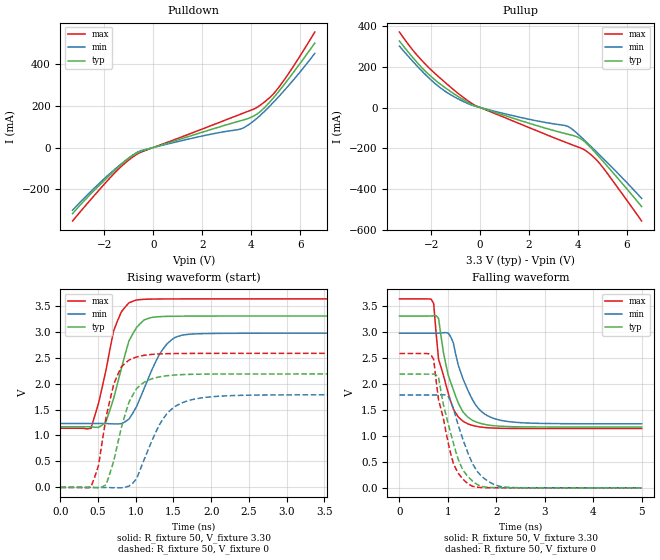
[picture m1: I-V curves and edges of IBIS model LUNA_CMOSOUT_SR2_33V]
[IBIS Ver]   3.2
[Comment Char]   |_char
[File name]   sg8201cja_33v_c.ibs
[File Rev]   1.1
[Date]   2021/10/19 9:35:58
[Source]
[Notes]
[Disclaimer]
This information is for modeling purposes only, and is not guaranteed.
Property of SEIKO EPSON Corp.,
unauthorized reproduction and/or distribution is strictly prohibited.
[Copyright]
Copyright 2021, SEIKO EPSON Corp.
[Component]   2G005_2016
Si_location Pin
Timing_location Pin
[Manufacturer]   SEIKO EPSON Corp.
| 2016 PKG
[Package]
R_pkg   25m   NA   NA
L_pkg   0.25n   NA   NA
C_pkg   0.183p   NA   NA
[Pin] signal_name   model_name
1   OE   NC
2   GND   GND
3   OUT   LUNA_CMOSOUT_SR2_33V
4   VCC   POWER
| Models and submodels in the file (1): LUNA_CMOSOUT_SR2_33V (Output)
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[Model]   LUNA_CMOSOUT_SR2_33V
Model_type Output
Polarity Non-Inverting
Vmeas=1.65
C_comp   2.5p   2.0p   3.0p
[Temperature Range] 25   140   -40
[Voltage Range]   3.30   2.97   3.63
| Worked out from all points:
|   slope of the pulldown table from 0 to 0.495 V, typ, clamps not added: 27.5 ohm
|   slope of the pullup table from 0 to 0.495 V, typ, clamps not added: 25.4 ohm
|   falling waveform, R_fixture 50, V_fixture 3.30: 20-80 % time 369ps typ, 437ps min, 324ps max; typ from 3.3 V to 1.17 V
|   falling waveform, R_fixture 50, V_fixture 0: 20-80 % time 385ps typ, 436ps min, 343ps max; typ from 2.19 V to 0 V
|   rising waveform, R_fixture 50, V_fixture 3.30: 20-80 % time 249ps typ, 325ps min, 229ps max; typ from 1.17 V to 3.3 V
|   rising waveform, R_fixture 50, V_fixture 0: 20-80 % time 256ps typ, 354ps min, 215ps max; typ from 0 V to 2.19 V
[Pullup]
-3.3V     326.6mA    301.4mA    370.6mA
-2.6V     224.1mA    206.5mA    259.7mA
-1.7V     121.2mA    103.6mA    151.2mA
-1.1V     69.8mA     55.27mA    88.8mA
-300mV    12.86mA    10.04mA    16.82mA
1.8V      -69.82mA   -52.54mA   -88.74mA
3.5V      -128.5mA   -89.13mA   -171.1mA
3.7V      -134.3mA   -100.9mA   -180.4mA
4V        -146.3mA   -131mA     -193.9mA
4.4V      -182.1mA   -176.3mA   -219.2mA
5V        -261mA     -246.9mA   -291.9mA
6.6V      -486.1mA   -446.4mA   -557.1mA
[Pulldown]
-3.3V     -315.7mA   -299.4mA   -351.1mA
-2.6V     -226.9mA   -215.5mA   -254.4mA
-1.6V     -112.3mA   -106.8mA   -123.8mA
-1.1V     -59.75mA   -58.96mA   -69.15mA
-700mV    -28.75mA   -25.32mA   -34.58mA
1.5V      54.78mA    42.07mA    65.84mA
3.6V      129mA      89.55mA    160.8mA
4.1V      150.4mA    126.4mA    183.3mA
4.5V      185.6mA    167.6mA    213.4mA
4.9V      235.9mA    214.7mA    254.9mA
5.3V      293.2mA    265.6mA    314.7mA
6.6V      498.9mA    449.6mA    551.8mA
[Falling Waveform]
R_fixture=50
V_fixture=3.30
V_fixture_min=2.97
V_fixture_max=3.63
0s        3.3V       2.97V      3.63V
707.1ps   3.304V     2.969V     3.537V
808.1ps   3.255V     2.97V      2.468V
909.1ps   2.595V     2.98V      2.16V
1.01ns    2.157V     2.971V     1.809V
1.162ns   1.757V     2.567V     1.437V
1.364ns   1.405V     1.981V     1.253V
1.667ns   1.24V      1.49V      1.17V
2.071ns   1.185V     1.302V     1.145V
5ns       1.168V     1.231V     1.139V
[Falling Waveform]
R_fixture=50
V_fixture=0
V_fixture_min=0
V_fixture_max=0
0s        2.185V     1.784V     2.581V
707.1ps   2.185V     1.783V     2.465V
808.1ps   2.116V     1.784V     1.686V
1.01ns    1.22V      1.755V     845.1mV
1.111ns   868.5mV    1.537V     475.4mV
1.313ns   339mV      923.7mV    166.5mV
1.465ns   168.9mV    558.7mV    50.75mV
1.717ns   23.77mV    205.3mV    5.662mV
2.121ns   3.009mV    21.88mV    1.362mV
5ns       280.9uV    482.4uV    182.3uV
[Rising Waveform]
R_fixture=50
V_fixture=3.30
V_fixture_min=2.97
V_fixture_max=3.63
0s        1.168V     1.231V     1.139V
404ps     1.167V     1.231V     1.138V
606.1ps   1.269V     1.23V      2.269V
707.1ps   1.719V     1.223V     3.02V
808.1ps   2.287V     1.228V     3.38V
909.1ps   2.821V     1.315V     3.554V
1.01ns    3.079V     1.557V     3.61V
1.313ns   3.288V     2.563V     3.627V
1.616ns   3.297V     2.932V     3.629V
5ns       3.3V       2.97V      3.63V
[Rising Waveform]
R_fixture=50
V_fixture=0
V_fixture_min=0
V_fixture_max=0
0s        0V         0V         0V
404ps     -682.4uV   187.3uV    7.435mV
505.1ps   -7.859mV   370.7uV    420.8mV
606.1ps   53.3mV     -838.1uV   1.356V
707.1ps   507mV      -5.814mV   1.985V
808.1ps   1.15V      -7.496mV   2.32V
1.01ns    1.902V     166.4mV    2.512V
1.364ns   2.14V      1.322V     2.573V
1.717ns   2.177V     1.68V      2.58V
5ns       2.185V     1.783V     2.581V
[Ramp]
R_load=50
dV/dt_r   1.311E+0/2.538E-10   1.070E+0/3.542E-10   1.549E+0/2.147E-10
dV/dt_f   1.279E+0/3.691E-10   1.044E+0/4.348E-10   1.494E+0/3.233E-10
|[End   LUNA_CMOSOUT_SR2_33V
